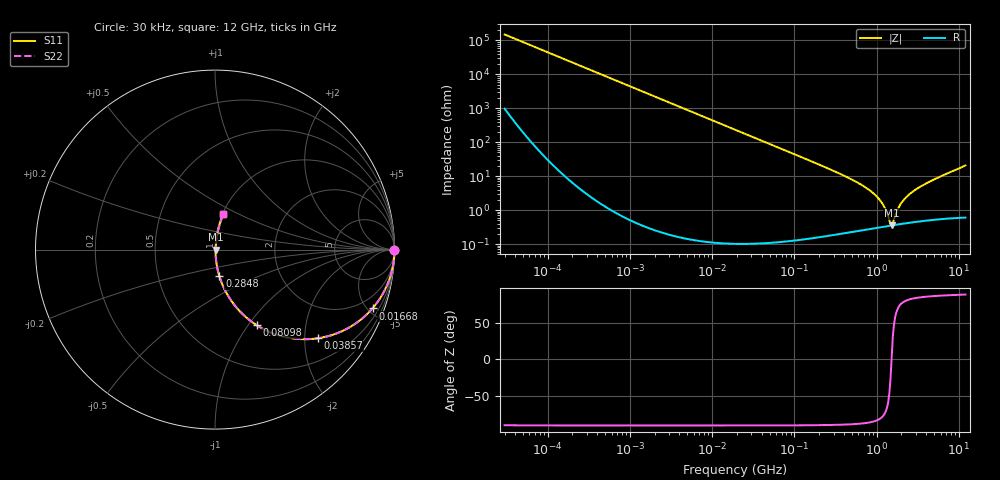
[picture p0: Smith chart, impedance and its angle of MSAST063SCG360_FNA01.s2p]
! MSAST063SCG360_FNA01  S-PARAMETER MODEL  ( Standard Model )
! Model Generated by TAIYO YUDEN Corporation (http://www.ty-top.com)
! Version 1.0
! TAIYO YUDEN Control No. 241122
! Copyright(c) 2024 TAIYO YUDEN CO.,LTD. All Rights Reserved.
! Product Description (link to TY-COMPAS)
! https://ds.yuden.co.jp/TYCOMPAS/or/detail?pn=MSAST063SCG360JFNA01&u=M
! Products Name : Multilayer Ceramic Capacitors
! Characteristics :
!  Capacitance : 36 [pF] , Rated Voltage : 25 [V] , TCC : CG / C0G
!  Case Size : 0.6 x 0.3 / 0.024 x 0.012 [mm/inch] , Thickness : 0.3 / 0.012 [mm/inch]
!  (Conditions: Temperature = 25 [degC] , DC Bias Voltage = 0 [V])
! External Node Assignments :
!  1  o---| |---o  2
! GND o---------o GND
! Frequency Range : 0.03MHz  -  12000MHz  [ 401 STEP ]
# MHZ S RI R 50
! Freq[MHz].  S11 Real  S11 Imag  S21 Real  S21 Imag  S12 Real  S12 Imag  S22 Real  S22 Imag
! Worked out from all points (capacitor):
!   401 points, 30 kHz to 12 GHz, reference 50 ohm
!   read as one part in series: C = 35.6 pF near 32 kHz
!   lowest |Z| = 356 mohm at 1.524 GHz (marker M1)
!   series resonance near 1.518 GHz, so ESL is about 310 pH
!   S11 on the Smith chart (normalised r, x): 30 kHz: open; 16.68 MHz: 1.00, -5.36; 38.57 MHz: 1.00, -2.32; 80.98 MHz: 1.00, -1.10; 284.8 MHz: 1.00, -0.30; 12 GHz: 1.01, +0.41
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0.03  1 -0.000671  4.84e-06 0.000671  4.84e-06 0.000671  1 -0.000671
0.260295  1 -0.00583  3.52e-05 0.00583  3.52e-05 0.00583  1 -0.00583
2.258455  0.9974 -0.0504  0.00255 0.0504  0.00255 0.0504  0.9974 -0.0504
6.54608  0.979 -0.1434  0.021 0.1434  0.021 0.1434  0.979 -0.1434
16.67749  0.8776 -0.3276  0.1224 0.3276  0.1224 0.3276  0.8776 -0.3276
18.97367  0.8471 -0.3597  0.1529 0.3597  0.1529 0.3597  0.8471 -0.3597
38.57132  0.5726 -0.4943  0.4274 0.4943  0.4274 0.4943  0.5726 -0.4943
80.98098  0.2328 -0.4216  0.7672 0.4216  0.7672 0.4216  0.2328 -0.4216
164.6252  0.0683 -0.2495  0.9317 0.2495  0.9317 0.2495  0.0683 -0.2495
284.8288  0.0241 -0.1474  0.9759 0.1474  0.9759 0.1474  0.0241 -0.1474
579.0248  0.00671 -0.0654  0.9933 0.0654  0.9933 0.0654  0.00671 -0.0654
909.4299  0.00388 -0.0313  0.9961 0.0313  0.9961 0.0313  0.00388 -0.0313
1177.092  0.00344 -0.0151  0.9966 0.0151  0.9966 0.0151  0.00344 -0.0151
1296.659  0.00342 -0.00929  0.9966 0.00929  0.9966 0.00929  0.00342 -0.00929
1428.372  0.00347 -0.0036  0.9965 0.0036  0.9965 0.0036  0.00347 -0.0036
1523.532  0.00354 0.000208  0.9965 -0.000208  0.9965 -0.000208  0.00354 0.000208
1625.032  0.00365 0.00394  0.9964 -0.00394  0.9964 -0.00394  0.00365 0.00394
1790.1  0.00385 0.00917  0.9962 -0.00917  0.9962 -0.00917  0.00385 0.00917
1971.936  0.00412 0.015  0.9959 -0.015  0.9959 -0.015  0.00412 0.015
2722.352  0.00552 0.0341  0.9945 -0.0341  0.9945 -0.0341  0.00552 0.0341
4710.119  0.0106 0.0734  0.9894 -0.0734  0.9894 -0.0734  0.0106 0.0734
12000  0.0465 0.1966  0.9535 -0.1966  0.9535 -0.1966  0.0465 0.1966
